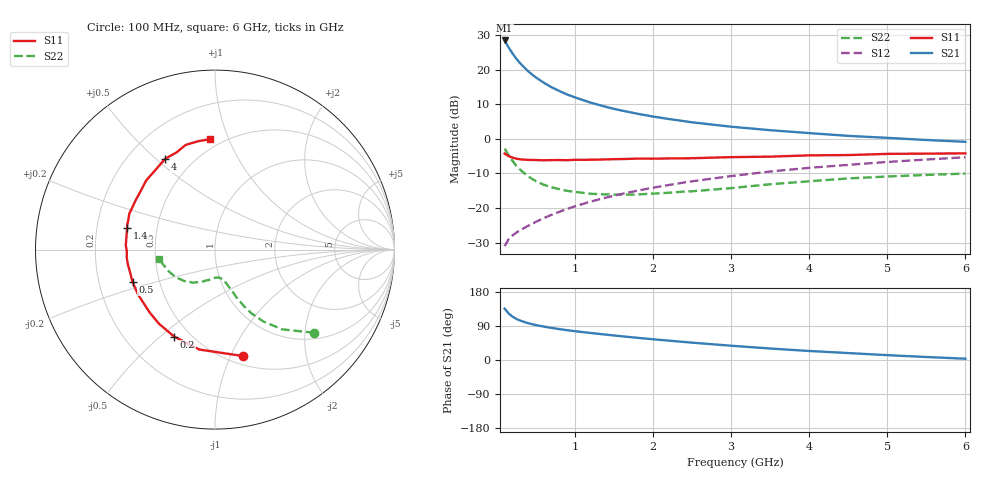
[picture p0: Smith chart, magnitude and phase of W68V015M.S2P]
! SIEMENS Small Signal Semiconductors
! BFR193W
! Si NPN RF Bipolar Junction Transistor in SOT323
! VCE = 8 V  IC = 15 mA
! Common Emitter S-Parameters:  September  1992
# GHz  S  MA  R  50
!  f  S11  S21  S12  S22
! GHz  MAG  ANG  MAG  ANG  MAG  ANG  MAG  ANG
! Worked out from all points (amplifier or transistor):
!   28 points, 100 MHz to 6 GHz, reference 50 ohm
!   highest |S21| = 28.4 dB at 100 MHz (marker M1)
!   |S21| within 3 dB of that: start of sweep to 179.6 MHz
!   unconditionally stable (mu >= 1): 875.7 MHz to 2.607 GHz
!   at 300 MHz: K = 0.67, MSG = 24.1 dB, |S12| = -26.4 dB
!   at 1.5 GHz: K = 1.04, MAG = 11.3 dB, |S12| = -16.4 dB
!   at 6 GHz: K = 0.90, MSG = 2.2 dB, |S12| = -5.3 dB
!   S11 on the Smith chart (normalised r, x): 100 MHz: 0.59, -1.11; 200 MHz: 0.41, -0.56; 500 MHz: 0.35, -0.17; 1.4 GHz: 0.33, +0.11; 4 GHz: 0.35, +0.54; 6 GHz: 0.43, +0.86
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0.1  0.613 -75.3  26.29 135.5  0.0282 60.5  0.7224 -39.9
0.15  0.5637 -98.9  20.98 123.0  0.0353 55.1  0.5819 -49.8
0.2  0.5354 -115.2  17.14 114.5  0.0401 53.1  0.4823 -56.1
0.25  0.5176 -127.2  14.34 108.5  0.0443 52.7  0.4075 -60.3
0.3  0.5052 -136.1  12.29 103.9  0.048 53.4  0.3578 -62.7
0.4  0.4966 -149.5  9.466 97.1  0.0554 55.7  0.2872 -66.0
0.5  0.4939 -158.4  7.691 92.2  0.0633 58.0  0.245 -67.8
0.6  0.4899 -165.1  6.469 88.2  0.0717 59.9  0.2176 -69.9
0.7  0.4925 -170.5  5.559 84.7  0.0798 61.5  0.1999 -71.1
0.8  0.4937 -175.0  4.903 81.5  0.0882 62.8  0.1877 -72.8
0.9  0.4913 -179.0  4.371 78.7  0.0972 63.6  0.1773 -73.8
1  0.4976 177.3  3.968 76.0  0.1061 64.2  0.1715 -75.4
1.2  0.4988 171.2  3.334 71.3  0.1239 65.0  0.1611 -79.3
1.4  0.5041 166.3  2.886 66.9  0.1417 65.1  0.1575 -82.8
1.8  0.5178 157.3  2.302 58.6  0.1785 64.4  0.1574 -90.9
2.2  0.5205 148.4  1.933 51.1  0.2153 63.0  0.1665 -98.0
3  0.5437 134.8  1.495 37.7  0.2898 58.4  0.1941 -112.6
3.5  0.5527 127.4  1.332 30.3  0.3374 54.7  0.2208 -123.5
4  0.577 118.8  1.209 23.8  0.3811 50.6  0.2436 -133.6
4.5  0.5828 111.4  1.103 18.3  0.4209 46.6  0.2681 -144.9
5.5  0.6113 98.7  0.961 7.9  0.5027 38.5  0.3008 -164.1
6  0.6161 92.5  0.905 3.4  0.5418 34.0  0.3148 -170.1
